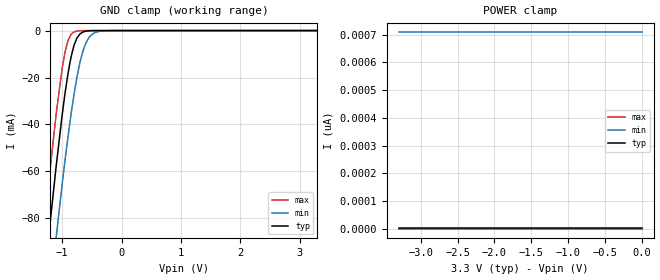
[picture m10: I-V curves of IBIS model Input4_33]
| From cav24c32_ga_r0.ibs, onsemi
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|//////////////////////////////////////////////////////////////////////////////
|//////////////////////////////////////////////////////////////////////////////
[Model]  Input4_33
Model_type Input
Vinh = 2.31
Vinl = 0.99
|  variable   typ   min   max
C_comp   6pF   6pF   6pF
|//////////////////////////////////////////////////////////////////////////////
[Temperature Range]   25   125   -40
|//////////////////////////////////////////////////////////////////////////////
[Voltage Range]   3.30V   3.00V   3.60V
|//////////////////////////////////////////////////////////////////////////////
[POWER Clamp Reference] 3.30V   3.00V   3.60V
|//////////////////////////////////////////////////////////////////////////////
[GND Clamp Reference]   0V   0V   0V
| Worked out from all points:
|   GND clamp passes 1 mA (typ) near -0.67 V on its own axis
|//////////////////////////////////////////////////////////////////////////////
[GND Clamp]
|   Voltage   I(typ)   I(min)   I(max)
-3.3V     -664mA     -675mA     -649mA
-1.4V     -132mA     -161mA     -109mA
-1.3V     -106mA     -136mA     -83.4mA
-1.2V     -81.3mA    -111mA     -58.4mA
-1.1V     -57.6mA    -87.8mA    -35.4mA
-950mV    -26.4mA    -54.9mA    -8.94mA
-900mV    -18.1mA    -45mA      -4.16mA
-800mV    -6.26mA    -27.2mA    -569uA
-700mV    -1.43mA    -13.5mA    -61.6uA
-600mV    -261uA     -5.28mA    -6.43uA
-400mV    -7.69uA    -463uA     -69.7nA
3.3V      4pA        708pA      35.2fA
|//////////////////////////////////////////////////////////////////////////////
[POWER Clamp]
|   Voltage   I(typ)   I(min)   I(max)
-3.3V     4pA        708pA      35.1fA
-600mV    4pA        708pA      35.1fA
-500mV    4pA        708pA      35.3fA
0V        4pA        708pA      35.3fA
